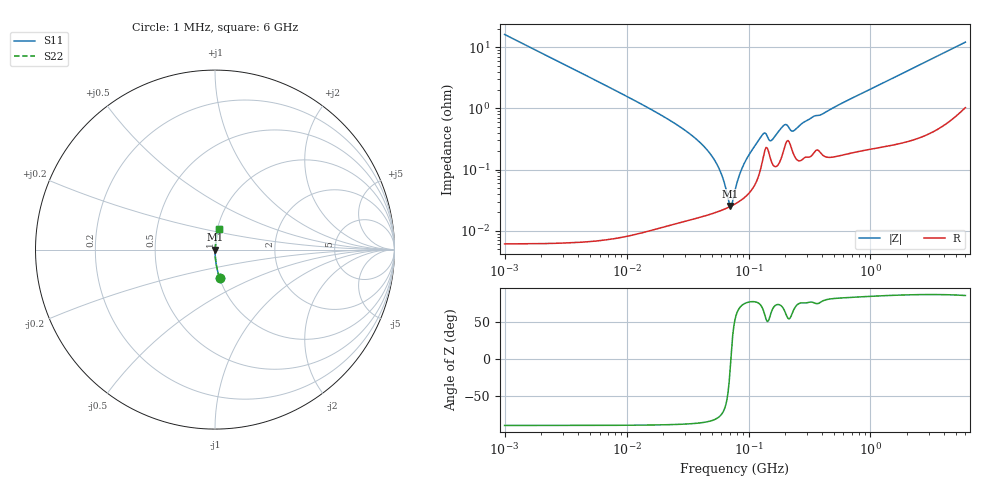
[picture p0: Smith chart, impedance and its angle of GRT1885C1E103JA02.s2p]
!Murata Part Number: GRT1885C1E103JA02
!These Parameters are Measured in Series Mode Connection
!Data Generated on Jun 19, 2026
!  o--ll--o
!Port1  Port2
!  o------o
!Operation Temp=25[degC], DC Bias Voltage=0[V]
!Freq. Start=1000[kHz] Stop=6[GHz] 401[Steps]
# Hz S RI R 50
!Freq.(Hz) S11(Real) S11(Imag) S21(Real) S21(Imag) S12(Real) S12(Imag) S22(Real) S22(Imag)
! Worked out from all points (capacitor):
!   401 points, 1 MHz to 6 GHz, reference 50 ohm
!   read as one part in series: C = 9.87 nF near 1.044 MHz
!   lowest |Z| = 25.4 mohm at 71.01 MHz (marker M1)
!   series resonance near 71.66 MHz, so ESL is about 500 pH
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1000000  0.0254 -0.1571  0.9746 0.1571  0.9746 0.1571  0.0254 -0.1571
4293785  0.00146 -0.0373  0.9985 0.0373  0.9985 0.0373  0.00146 -0.0373
1.843659e7  0.000176 -0.00813  0.9998 0.00813  0.9998 0.00813  0.000176 -0.00813
3.245342e7  0.000164 -0.00394  0.9998 0.00394  0.9998 0.00394  0.000164 -0.00394
4.697123e7  0.000187 -0.00196  0.9998 0.00196  0.9998 0.00196  0.000187 -0.00196
5.838291e7  0.000213 -0.000937  0.9998 0.000937  0.9998 0.000937  0.000213 -0.000937
6.23192e7  0.000223 -0.000638  0.9998 0.000638  0.9998 0.000638  0.000223 -0.000638
6.798347e7  0.00024 -0.000241  0.9998 0.000241  0.9998 0.000241  0.00024 -0.000241
7.100585e7  0.000251 -4.18e-05  0.9997 4.18e-05  0.9997 4.18e-05  0.000251 -4.18e-05
7.416259e7  0.000262 0.000159  0.9997 -0.000159  0.9997 -0.000159  0.000262 0.000159
7.745967e7  0.000275 0.000361  0.9997 -0.000361  0.9997 -0.000361  0.000275 0.000361
8.450008e7  0.000306 0.000776  0.9997 -0.000776  0.9997 -0.000776  0.000306 0.000776
9.218041e7  0.000349 0.00121  0.9997 -0.00121  0.9997 -0.00121  0.000349 0.00121
1.305463e8  0.00144 0.00346  0.9986 -0.00346  0.9986 -0.00346  0.00144 0.00346
1.363501e8  0.0021 0.00336  0.9979 -0.00336  0.9979 -0.00336  0.0021 0.00336
1.553559e8  0.0013 0.00274  0.9987 -0.00274  0.9987 -0.00274  0.0013 0.00274
1.973453e8  0.00233 0.00485  0.9977 -0.00485  0.9977 -0.00485  0.00233 0.00485
2.348496e8  0.00177 0.00393  0.9982 -0.00393  0.9982 -0.00393  0.00177 0.00393
3.325952e8  0.00177 0.00693  0.9982 -0.00693  0.9982 -0.00693  0.00177 0.00693
4.045054e8  0.00179 0.0079  0.9982 -0.0079  0.9982 -0.0079  0.00179 0.0079
1.428092e9  0.00329 0.029  0.9967 -0.029  0.9967 -0.029  0.00329 0.029
6e9  0.024 0.1163  0.976 -0.1163  0.976 -0.1163  0.024 0.1163
